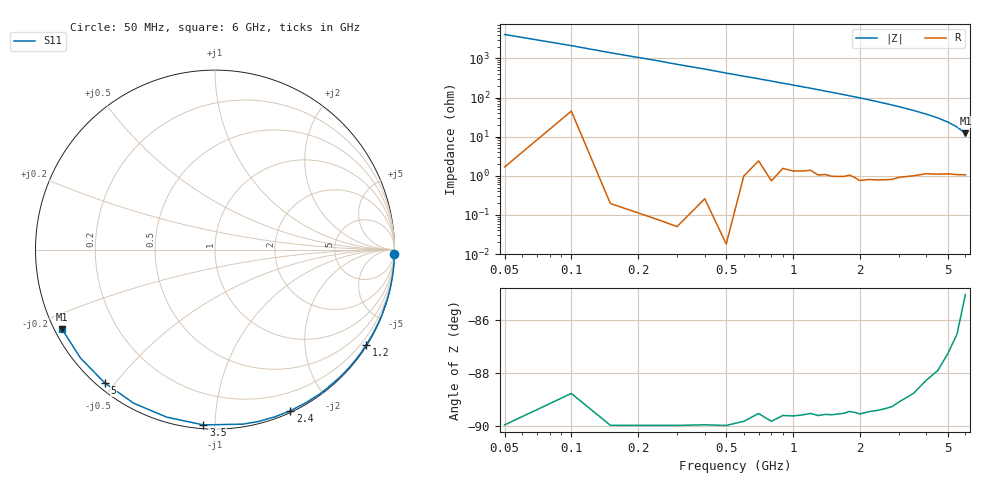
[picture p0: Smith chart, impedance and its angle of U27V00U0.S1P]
! SIEMENS Discrete & RF Semiconductors
! BBY52-02W
! Si Tuning Diode in SCD-80
! VR = 7 V
! S-Parameters:  September  1997
# GHz  S  MA  R  50
!  f  S11
! GHz  MAG  ANG
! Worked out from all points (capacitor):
!   34 points, 50 MHz to 6 GHz, reference 50 ohm
!   read as one part to ground: C = 760 fF near 50 MHz
!   lowest |Z| = 12.2 ohm at 6 GHz (marker M1)
!   S11 on the Smith chart (normalised r, x): 50 MHz: 0, -82; 1.2 GHz: 0.03, -3.45; 2.4 GHz: 0.02, -1.57; 3.5 GHz: 0.02, -0.94; 5 GHz: 0.02, -0.47; 6 GHz: 0.02, -0.24
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0.05  1 -1.4
0.25  1 -6.7
0.3  1 -8.1
0.4  0.9999 -10.7
0.5  1 -13.5
0.6  0.9992 -16.2
0.8  0.999 -21.5
0.9  0.9973 -24.3
1  0.9971 -26.9
1.1  0.9966 -29.6
1.2  0.9957 -32.3
1.3  0.9962 -35.0
1.4  0.9955 -37.8
1.6  0.9948 -43.2
1.7  0.9942 -45.8
1.8  0.993 -48.6
2  0.9938 -54.0
2.2  0.9921 -59.5
2.4  0.991 -64.9
2.6  0.9896 -70.3
2.8  0.9879 -75.7
3  0.9848 -80.9
3.5  0.9789 -93.8
4  0.9715 -106.1
4.5  0.9683 -117.8
5  0.9639 -129.5
5.5  0.9626 -141.1
6  0.9608 -152.6
